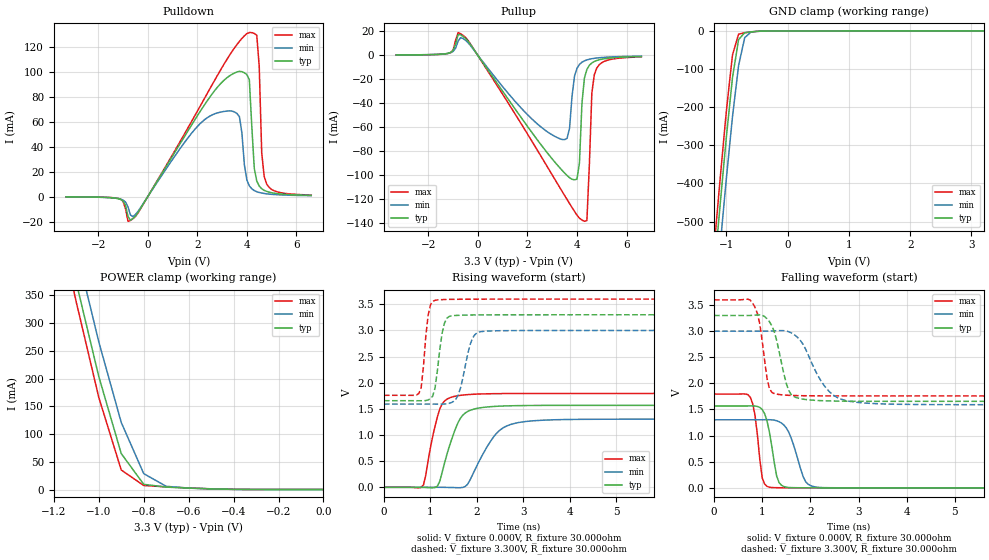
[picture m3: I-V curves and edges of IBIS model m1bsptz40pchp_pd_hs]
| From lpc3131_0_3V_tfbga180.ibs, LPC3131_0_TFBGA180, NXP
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| |   Rev 0.20 IBIS Model Design Automation Generation   |
| |   N O N - S I L I C O N   C O R R E L A T E D   |
| |   This IBIS [Model] is pre-Beta tactical support   |
| |  Note: this IBIS [Model] contains clamp curves generated   |
| |   through simulation which should not be relied upon   |
| Date/Time   : 2010 Jan 25 (Mon) 11:58:19
| Pccmos090 jliolib_p50 2.0
|   0.9 um 3.3V pad library
|   seven level metal
|   dual oxide
|   dual threshold voltage
|   nominal line mixed supply
|   parasitic extracted netlists
| Process block a10
| mem1bsptz40pchp
|   Bidirectional Pad 3.3
|   3state Output
|   Plain Input
|   CMOS
|   Programmable between
|   - (p1=0, p2=1) plain input
|   - (p1=0, p2=0) with Pull Up
|   - (p1=1, p2=1) with Pull Down
|   - (p1=1, p2=0) with Repeater
| Pull Down Mode high speed(esh=0, p1=1, p2=1)
[Model]   m1bsptz40pchp_pd_hs | of mem1bsptz40pchp
Model_type   I/O
Polarity   Non-Inverting
Enable   Active-Low
|  Reciever Thresholds
Vinl   = 0.99V
Vinh   = 2.31V
| AC Test Load Conditions
Vref   = 0
Cref   = 0
Rref   = 1000000000
Vmeas   = 1.65
| [Process Range]   typical   min   max
| C_comp edge width   400.000ps   400.000ps   400.000ps
| C_comp Tstrobe   40.000fs   40.000fs   40.000fs
C_comp   200.000pF   200.000pF   200.000pF
[Temperature Range]   25   125   -40
[Voltage Range]   3.30V   3.00V   3.60V
[GND Clamp Reference]   0.00V   0.00V   0.00V
[Pulldown Reference]   0.00V   0.00V   0.00V
[POWER Clamp Reference]   3.30V   3.00V   3.60V
[Pullup Reference]   3.30V   3.00V   3.60V
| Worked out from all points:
|   slope of the pulldown table from 0 to 0.495 V, typ, clamps not added: 30.9 ohm
|   slope of the pullup table from 0 to 0.495 V, typ, clamps not added: 33.2 ohm
|   GND clamp passes 1 mA (typ) near -0.51 V on its own axis
|   POWER clamp passes 1 mA (typ) near -0.45 V on its own axis
|   rising waveform, V_fixture 0.000V, R_fixture 30.000ohm: 20-80 % time 343ps typ, 517ps min, 257ps max; typ from 0 V to 1.57 V
|   falling waveform, V_fixture 0.000V, R_fixture 30.000ohm: 20-80 % time 177ps typ, 272ps min, 137ps max; typ from 1.57 V to 0 V
|   rising waveform, V_fixture 3.300V, R_fixture 30.000ohm: 20-80 % time 145ps typ, 213ps min, 116ps max; typ from 1.66 V to 3.3 V
|   falling waveform, V_fixture 3.300V, R_fixture 30.000ohm: 20-80 % time 249ps typ, 498ps min, 169ps max; typ from 3.3 V to 1.66 V
[GND Clamp]
| ref voltage   0.00V   0.00V   0.00V
|   Voltage   I(typ)   I(min)   I(max)
-3.3V     -4.732A    -4.814A    -4.684A
-1.2V     -636mA     -742.5mA   -569.7mA
-1.1V     -453.5mA   -561.8mA   -385.7mA
-1V       -279mA     -387.5mA   -210.8mA
-900mV    -122.8mA   -225.5mA   -63.13mA
-800mV    -22.45mA   -90.49mA   -8.204mA
-700mV    -4.394mA   -17.31mA   -4.534mA
-600mV    -2.163mA   -3.055mA   -2.529mA
-300mV    -78.17uA   -69.01uA   -98.11uA
3.2V      308.4uA    167.8uA    522.1uA
[Power Clamp]   | Vtable = Vcc - Vpad
| ref voltage   3.30V   3.00V   3.60V
|   Voltage   I(typ)   I(min)   I(max)
-3.3V     4.647A     4.675A     4.636A
-1.2V     553.3mA    610.4mA    520.8mA
-1.1V     373.2mA    433.6mA    337.9mA
-1V       204.1mA    266.6mA    166.5mA
-900mV    65.1mA     121.2mA    35.47mA
-800mV    9.693mA    28.95mA    7.599mA
-700mV    4.658mA    6.108mA    5.079mA
-600mV    2.822mA    2.869mA    3.125mA
-400mV    573.3uA    634.5uA    703uA
0V        308.5uA    161.6uA    522.8uA
[Pulldown]
| ref voltage   0.00V   0.00V   0.00V
|   Voltage   I(typ)   I(min)   I(max)
-3.3V     -236.7uA   -252.6uA   -192uA
-1.2V     -1.652mA   -1.556mA   -1.496mA
-600mV    -17.54mA   -16.01mA   -17.75mA
2.9V      89.5mA     67.39mA    99.97mA
3.7V      100.2mA    63.94mA    124.2mA
4.1V      93.4mA     8.546mA    131.2mA
4.3V      22.52mA    4.759mA    130.5mA
4.4V      12.45mA    3.873mA    129.1mA
4.5V      8.402mA    3.255mA    104mA
4.6V      6.246mA    2.801mA    34.93mA
4.8V      4.127mA    2.184mA    10.1mA
6.6V      979.6uA    712.7uA    1.221mA
[Pullup]   | Vtable = Vcc - Vpad
| ref voltage   3.30V   3.00V   3.60V
|   Voltage   I(typ)   I(min)   I(max)
-3.3V     207.2uA    209.5uA    174.1uA
-500mV    13.97mA    12.41mA    14.82mA
3.4V      -96.32mA   -70.52mA   -113.9mA
3.7V      -102.5mA   -61.11mA   -124.1mA
3.9V      -104.2mA   -17.59mA   -130.7mA
4.1V      -89.97mA   -7.665mA   -136.3mA
4.2V      -40.47mA   -5.865mA   -137.9mA
4.3V      -19.14mA   -4.724mA   -138.9mA
4.4V      -11.89mA   -3.942mA   -138.3mA
4.6V      -6.502mA   -2.948mA   -31.69mA
4.7V      -5.28mA    -2.614mA   -16.33mA
6.6V      -1.118mA   -810uA     -1.413mA
[Ramp]
R_load   = 30.000ohm
|   dV/dt(typ)   dV/dt(min)   dV/dt(max)
dV/dt_r   940.471mV/350.000ps   781.939mV/500.000ps   1.077V/250.000ps
dV/dt_f   985.826mV/250.000ps   844.548mV/500.000ps   1.103V/150.000ps
[Rising Waveform]  | cubic spline decimation from 501 points
V_fixture   = 0.000V
R_fixture   = 30.000ohm
|   Time   V(typ)   V(min)   V(max)
0s        3.993nV    181.6nV    2.818nV
850ps     -1.566mV   23.17uV    44.27mV
1.15ns    23.74mV    142.8uV    1.35V
1.35ns    615.7mV    -1.771mV   1.683V
1.6ns     1.249V     -8.251mV   1.752V
1.75ns    1.422V     16.92mV    1.769V
2.45ns    1.55V      1.058V     1.791V
2.75ns    1.559V     1.208V     1.793V
3.35ns    1.565V     1.28V      1.795V
25ns      1.567V     1.303V     1.795V
[Falling Waveform]  | cubic spline decimation from 501 points
V_fixture   = 0.000V
R_fixture   = 30.000ohm
|   Time   V(typ)   V(min)   V(max)
0s        1.567V     1.303V     1.795V
750ps     1.569V     1.303V     1.738V
850ps     1.566V     1.303V     1.388V
1ns       1.5V       1.303V     190.9mV
1.2ns     786.7mV    1.302V     6.195mV
1.3ns     223.6mV    1.285V     3.131mV
1.4ns     49.89mV    1.24V      1.81mV
1.9ns     1.221mV    120.2mV    236.1uV
2.2ns     449.4uV    7.242mV    87.38uV
25ns      15.51nV    225.5nV    -36.29nV
[Rising Waveform]  | cubic spline decimation from 501 points
V_fixture   = 3.300V
V_fixture_min = 3.000V
V_fixture_max = 3.600V
R_fixture   = 30.000ohm
|   Time   V(typ)   V(min)   V(max)
0s        1.656V     1.591V     1.759V
750ps     1.655V     1.591V     1.791V
800ps     1.655V     1.591V     1.903V
950ps     1.67V      1.591V     3.285V
1.15ns    2.234V     1.59V      3.583V
1.35ns    3.229V     1.596V     3.592V
1.6ns     3.288V     1.772V     3.595V
1.9ns     3.295V     2.84V      3.597V
2.2ns     3.297V     2.986V     3.598V
25ns      3.299V     2.999V     3.598V
[Falling Waveform]  | cubic spline decimation from 501 points
V_fixture   = 3.300V
V_fixture_min = 3.000V
V_fixture_max = 3.600V
R_fixture   = 30.000ohm
|   Time   V(typ)   V(min)   V(max)
0s        3.299V     2.999V     3.598V
800ps     3.302V     2.999V     3.537V
950ps     3.311V     2.999V     3.132V
1.15ns    3.178V     3.001V     1.895V
1.25ns    2.989V     3.005V     1.805V
1.45ns    2.179V     3.008V     1.777V
1.65ns    1.752V     2.941V     1.767V
2.45ns    1.663V     1.794V     1.76V
3.15ns    1.657V     1.622V     1.759V
25ns      1.656V     1.591V     1.759V
